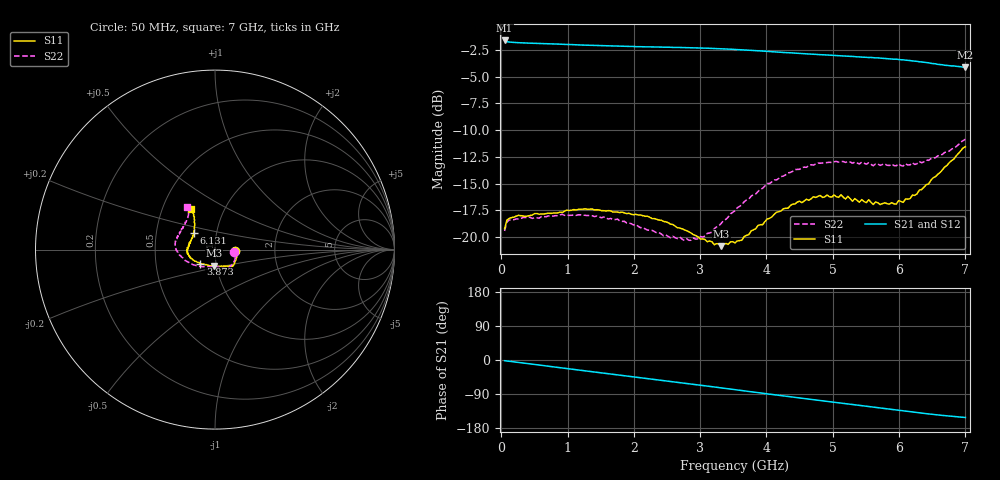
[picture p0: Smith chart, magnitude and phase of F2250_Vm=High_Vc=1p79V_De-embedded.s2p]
! Integrated Device Technology
! Corporate Headquarters
! 6024 Silver Creek Valley Road
! San Jose, CA 95138  USA
! Phone:  1-408-284-8200
! Toll Free:  1-800-223-1366
! Webpage:  http://www.idt.com/
! Timing and RF Division
! 515 Groton Road, Suite 102
! Westford, MA 01886-6024
! Device:  F2250
! Description: Voltage Variable RF Attenuator
! Frequency:  50.0 -  6000.00 MHz
! Package:  3x3 mm Thin QFN Plastic Package: 16 pin
! Ports:  2 RF, 3 DC
!  Pin  1  = GND
!  Pin  2  = NC
!  Pin  3  = RF1  = Port 1
!  Pin  4  = NC
!  Pin  5  = GND
!  Pin  6  = GND
!  Pin  7  = GND
!  Pin  8  = GND
!  Pin  9  = NC
!  Pin 10  = RF2  = Port 2
!  Pin 11  = NC
!  Pin 12  = GND
!  Pin 13  = GND
!  Pin 14  = VCNTRL
!  Pin 15  = VDD
!  Pin 16  = VMODE
! Vcntrl:  1.790 Volts
! Vmode:  +3.300 Volts
! Vdd:  +3.30  Volts
! Current:  1.325 mA
! Data:  The device was measured on a the F2250 evaluation board which has
!  individual transmission lines to the RF pins.  Data was collected
!  using a calibrated network analyzer.  The evaluation board was
!  de-embedded using a TRL calibration technique.
!  The reference plane is the edge of the package pin.
! Misc:  SN 10
!  Action Tracker AT0258
! Date Measured:  2014-11-26
! Date:  2015-10-15  MJV
! Note:
!  Integrated Device Technology supplies this data as a sample of measured
!  data at the package pin for this product.  Your particular data for this
!  product may vary.
!  Data was taken at 25 degrees C.
!  Integrated Device Technology reserves the right to change this data at anytime.
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# GHz S dB R 50
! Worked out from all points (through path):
!   201 points, 50 MHz to 7 GHz, reference 50 ohm
!   highest |S21| = -1.60 dB at 50 MHz (marker M1); lowest = -4.1 dB at 7 GHz (marker M2)
!   group delay of S21, straight-line fit = 61 ps
!   lowest |S11| = -20.9 dB at 3.317 GHz (marker M3), VSWR 1.20, Z = 48.6 - j8.86 ohm
!   |S11| at or under -10 dB: start of sweep to end of sweep
!   |S22| runs from -20.3 to -10.9 dB; largest |S21 - S12| = 0.0018
!   S11 on the Smith chart (normalised r, x): 50 MHz: 1.24, -0.02; 3.873 GHz: 0.84, -0.13; 6.131 GHz: 0.78, +0.15; 7 GHz: 0.70, +0.34
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0.05  -19.23 -4.9  -1.60 -1.9  -1.60 -1.9  -19.45 -6.3
0.08475  -18.43 -4.8  -1.71 -2.5  -1.71 -2.5  -18.59 -5.9
0.1195  -18.27 -5.5  -1.75 -3.3  -1.75 -3.3  -18.42 -6.1
0.71025  -17.78 -25.6  -1.91 -16.5  -1.90 -16.5  -18.03 -31.0
1.2315  -17.40 -39.5  -2.03 -27.9  -2.03 -27.9  -17.96 -50.1
1.75275  -17.68 -46.5  -2.13 -39.0  -2.13 -39.1  -18.34 -61.1
2.37825  -18.43 -50.1  -2.21 -52.6  -2.22 -52.6  -19.60 -72.7
2.86475  -19.65 -62.2  -2.28 -63.4  -2.28 -63.4  -20.32 -94.8
3.07325  -20.25 -73.9  -2.32 -68.1  -2.31 -68.1  -19.93 -108.7
3.3165  -20.87 -93.6  -2.37 -73.6  -2.38 -73.6  -18.74 -125.2
3.525  -20.56 -110.9  -2.44 -78.3  -2.43 -78.4  -17.55 -137.1
3.8725  -18.93 -136.3  -2.56 -86.2  -2.56 -86.2  -15.75 -154.5
4.4285  -16.92 -160.7  -2.78 -98.5  -2.78 -98.5  -13.69 -173.8
4.7065  -16.25 -169.7  -2.89 -104.7  -2.88 -104.7  -13.27 179.4
5.1235  -16.06 179.5  -3.04 -113.8  -3.03 -113.8  -12.95 169.5
5.29725  -16.67 173.8  -3.09 -117.5  -3.10 -117.6  -13.10 166.1
5.332  -16.41 172.7  -3.12 -118.3  -3.11 -118.4  -13.00 165.2
5.61  -16.97 164.9  -3.21 -124.3  -3.20 -124.4  -13.33 158.5
5.85325  -16.93 154.1  -3.31 -129.6  -3.32 -129.7  -13.31 151.3
6.13125  -16.46 141.6  -3.46 -135.6  -3.47 -135.7  -13.27 143.7
6.54825  -14.36 127.3  -3.78 -144.3  -3.79 -144.4  -12.58 130.1
7  -11.56 120.1  -4.11 -151.7  -4.12 -151.8  -10.85 123.3
